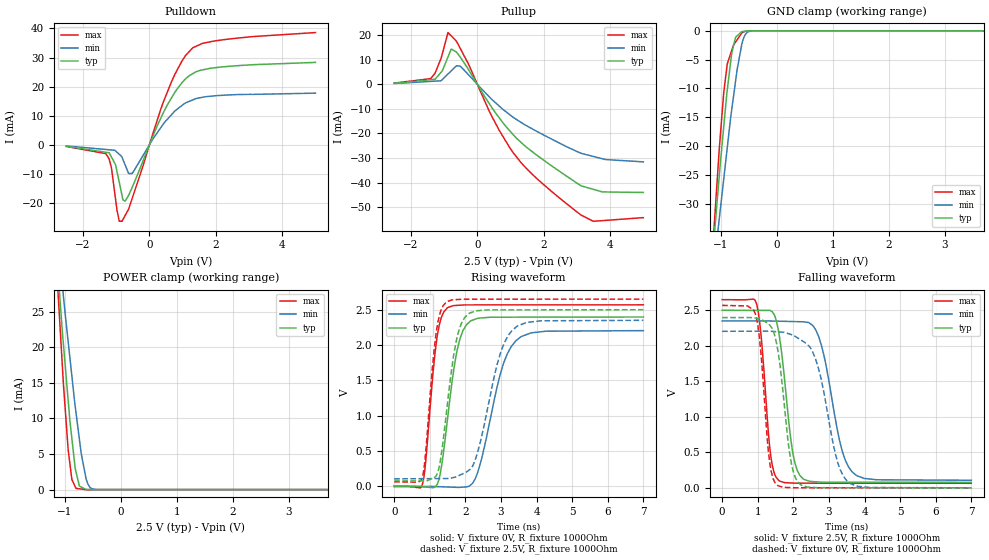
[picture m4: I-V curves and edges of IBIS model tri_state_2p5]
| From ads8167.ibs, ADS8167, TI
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|   tri_state_2p5 Model
[Model]   tri_state_2p5
Model_type   3-state
Polarity   Non-Inverting
Vmeas = 1.25
Vref = 0
Cref = 2pF
Rref = 100000
|   typ   min   max
C_comp   1.2590E-12F   1.2349E-12F  1.2624E-12F
|  Where Nom  PVT is Nominal Process, 2.5V,   27C
|   Fast PVT is Strong Process,  2.65V,  -40C
|   Slow PVT is Weak Process,   2.35V, 125C
[Voltage Range]   2.5   2.35   2.65
|Junction Temperature
[Temperature Range]   27   125   -40
[Pullup Reference]   2.5   2.35   2.65
[Pulldown Reference]   0   0   0
[Power Clamp Reference]   2.5   2.35   2.65
[GND Clamp Reference]   0   0   0
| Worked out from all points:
|   slope of the pulldown table from 0 to 0.375 V, typ, clamps not added: 37.8 ohm
|   slope of the pullup table from 0 to 0.375 V, typ, clamps not added: 45.9 ohm
|   GND clamp passes 1 mA (typ) near -0.72 V on its own axis
|   POWER clamp passes 1 mA (typ) near -0.76 V on its own axis
|   falling waveform, V_fixture 2.5V, R_fixture 1000Ohm: 20-80 % time 323ps typ, 514ps min, 240ps max; typ from 2.5 V to 0.078 V
|   rising waveform, V_fixture 0V, R_fixture 1000Ohm: 20-80 % time 381ps typ, 608ps min, 276ps max; typ from 0 V to 2.4 V
|   rising waveform, V_fixture 2.5V, R_fixture 1000Ohm: 20-80 % time 373ps typ, 613ps min, 268ps max; typ from 0.078 V to 2.5 V
|   falling waveform, V_fixture 0V, R_fixture 1000Ohm: 20-80 % time 330ps typ, 545ps min, 241ps max; typ from 2.4 V to 0 V
[Pulldown]
|   Voltage   I(typ)   I(min)   I(max)
-2.5V     -484.2uA   -349.2uA   -516.8uA
-1.31V    -2.518mA   -1.561mA   -2.984mA
-1.14V    -4.171mA   -1.733mA   -7.87mA
-1.017V   -6.807mA   -2.068mA   -18.7mA
-905.7mV  -12.81mA   -3.198mA   -26.21mA
-823.1mV  -17.28mA   -4.207mA   -26.23mA
-728.8mV  -19.31mA   -6.868mA   -24.26mA
-517.9mV  -14.63mA   -9.806mA   -18.42mA
231.9mV   6.449mA    4.101mA    8.302mA
660.4mV   16.03mA    10.3mA     21.55mA
1.303V    24.46mA    15.46mA    33.32mA
5V        28.35mA    17.79mA    38.6mA
[GND Clamp]
|   Voltage   I(typ)   I(min)   I(max)
-2.5V     -208.5mA   -173.2mA   -255.8mA
-1.174V   -42.12mA   -45.2mA    -42mA
-1.031V   -25.41mA   -32.85mA   -20.88mA
-947.6mV  -16.57mA   -25.65mA   -10.61mA
-884.8mV  -10.22mA   -20.24mA   -5.713mA
-805.7mV  -3.874mA   -13.69mA   -3.406mA
-735.7mV  -1.098mA   -8.646mA   -1.927mA
-710.5mV  -880uA     -6.832mA   -1.572mA
-625mV    -139.8uA   -2.315mA   -364.3uA
-551.5mV  -51.96uA   -489.7uA   -71.06uA
-437.5mV  -1.427uA   -21.82uA   -2.802uA
5V        0A         0A         0A
[Pullup]
|   Voltage   I(typ)   I(min)   I(max)
-2.5V     379.7uA    272.7uA    438.5uA
-1.4V     1.821mA    1.144mA    2.273mA
-1.084V   4.909mA    1.487mA    10.71mA
-881.6mV  11.05mA    4.135mA    20.97mA
-783.7mV  14.29mA    5.417mA    19.63mA
-517.9mV  11.1mA     7.354mA    14.7mA
660.4mV   -13.63mA   -8.883mA   -18.7mA
1.075V    -20.43mA   -13.39mA   -27.69mA
1.625V    -27.09mA   -17.92mA   -36.18mA
3.125V    -41.28mA   -28.07mA   -53.18mA
3.495V    -42.71mA   -29.35mA   -55.69mA
5V        -43.99mA   -31.55mA   -54.2mA
[POWER Clamp]
|   Voltage   I(typ)   I(min)   I(max)
-2.5V     188mA      156.8mA    229.4mA
-1.195V   37.89mA    40.42mA    37.05mA
-1.045V   21.94mA    28.47mA    17.04mA
-1.027V   20.28mA    27.05mA    14.65mA
-943.4mV  12.52mA    20.78mA    5.58mA
-877.7mV  7.19mA     15.98mA    1.434mA
-805.2mV  2.549mA    10.91mA    172.6uA
-743.2mV  500.2uA    7.089mA    113.4uA
-624.9mV  7.725uA    1.571mA    328.8nA
-563.6mV  4.293uA    426.8uA    281.8nA
-480.4mV  37.25nA    44.93uA    217.9nA
5V        0A         0A         0A
[Ramp]
R_load = 1000
|   typ   min   max
dV/dt_r   1.43833/3.80222e-10   1.32258/6.07345e-10   1.54165/2.74628e-10
dV/dt_f   1.45339/3.21356e-10   1.34581/5.11279e-10   1.55118/2.39347e-10
[Falling Waveform]
V_fixture = 2.5V
V_fixture_min = 2.35V
V_fixture_max = 2.65V
R_fixture = 1000Ohm
C_fixture = 0F
|   Time   V(typ)   V(min)   V(max)
0s        2.5V       2.35V      2.65V
963.3ps   2.498V     2.35V      2.598V
1.357ns   2.495V     2.349V     485.1mV
1.597ns   2.165V     2.347V     101.8mV
1.986ns   494.5mV    2.342V     67.52mV
2.276ns   126.7mV    2.338V     66.04mV
2.714ns   82.76mV    2.127V     65.91mV
3.303ns   80.01mV    660mV      65.75mV
3.643ns   79.8mV     230.4mV    65.65mV
7ns       77.69mV    106.9mV    64.71mV
[Rising Waveform]
V_fixture = 0V
V_fixture_min = 0V
V_fixture_max = 0V
R_fixture = 1000Ohm
C_fixture = 0F
|   Time   V(typ)   V(min)   V(max)
0s        4.926uV    107.4uV    -80.23nV
788.4ps   -7.197mV   3.266uV    23.27mV
1.194ns   18.38mV    -2.814mV   2.076V
1.487ns   909.5mV    -8.421mV   2.524V
1.758ns   1.902V     -13.59mV   2.561V
2.026ns   2.285V     -7.178mV   2.568V
2.384ns   2.381V     260.3mV    2.568V
3.083ns   2.395V     1.756V     2.568V
3.553ns   2.395V     2.115V     2.568V
7ns       2.397V     2.204V     2.569V
[Rising Waveform]
V_fixture = 2.5V
V_fixture_min = 2.35V
V_fixture_max = 2.65V
R_fixture = 1000Ohm
C_fixture = 0F
|   Time   V(typ)   V(min)   V(max)
0s        77.69mV    107mV      64.71mV
788.4ps   76.76mV    109.1mV    126.3mV
1.174ns   146.8mV    110.2mV    2.155V
1.467ns   1.044V     110.9mV    2.609V
1.728ns   2.02V      133.6mV    2.643V
1.976ns   2.387V     189.5mV    2.649V
2.335ns   2.486V     469.1mV    2.649V
3.003ns   2.498V     1.913V     2.649V
3.453ns   2.498V     2.266V     2.649V
7ns       2.5V       2.35V      2.65V
[Falling Waveform]
|Gnd
V_fixture = 0V
V_fixture_min = 0V
V_fixture_max = 0V
R_fixture = 1000Ohm
C_fixture = 0F
|   Time   V(typ)   V(min)   V(max)
0s        2.397V     2.204V     2.569V
936ps     2.39V      2.205V     2.448V
1.084ns   2.379V     2.206V     1.929V
1.327ns   2.298V     2.206V     391.3mV
1.557ns   1.957V     2.197V     35.1mV
1.936ns   369mV      2.16V      2.868mV
2.206ns   44.8mV     2.085V     1.263mV
2.624ns   4.68mV     1.815V     1.153mV
3.493ns   1.971mV    107.4mV    924.1uV
7ns       4.951uV    107.1uV    -233nV
